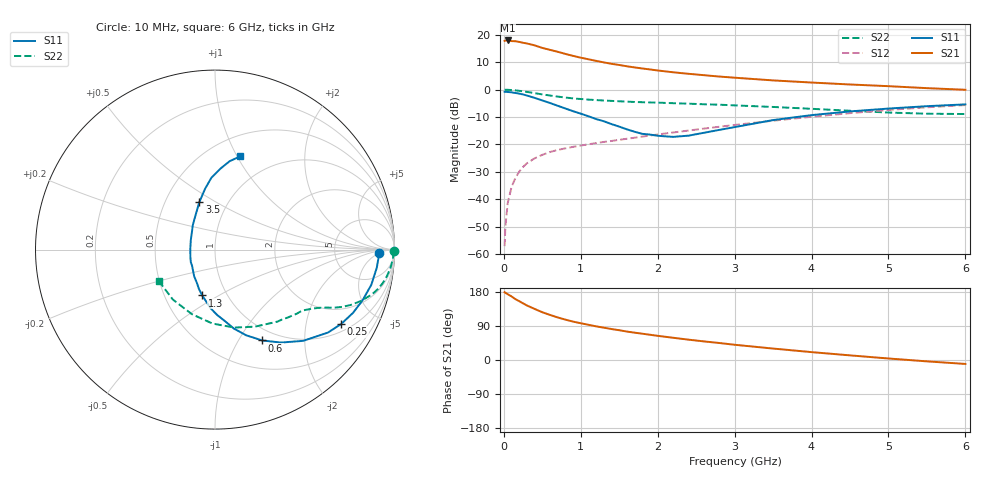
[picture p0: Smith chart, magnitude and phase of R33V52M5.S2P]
! SIEMENS Small Signal Semiconductors
! BFR181
! Si NPN RF Bipolar Junction Transistor in SOT23
! VCE = 3.5 V  IC = 2.5 mA
! Common Emitter S-Parameters:  May  1996
# GHz  S  MA  R  50
!  f  S11  S21  S12  S22
! GHz  MAG  ANG  MAG  ANG  MAG  ANG  MAG  ANG
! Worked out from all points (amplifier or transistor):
!   36 points, 10 MHz to 6 GHz, reference 50 ohm
!   highest |S21| = 17.9 dB at 50 MHz (marker M1)
!   |S21| within 3 dB of that: start of sweep to 539.6 MHz
!   unconditionally stable (mu >= 1): 1.481 GHz to 3.267 GHz
!   at 250 MHz: K = 0.27, MSG = 22.6 dB, |S12| = -28.2 dB
!   at 1.4 GHz: K = 0.98, MSG = 14.1 dB, |S12| = -18.7 dB
!   at 6 GHz: K = 0.86, MSG = 2.8 dB, |S12| = -5.6 dB
!   S11 on the Smith chart (normalised r, x): 10 MHz: 20, -5; 250 MHz: 1.29, -3.19; 600 MHz: 0.84, -1.26; 1.3 GHz: 0.77, -0.42; 3.5 GHz: 0.74, +0.42; 6 GHz: 0.70, +1.03
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0.01  0.9119 -1.3  7.759 178.8  0.0014 87.9  0.9964 -0.6
0.02  0.9127 -2.6  7.836 177.3  0.0032 86.0  0.9944 -1.3
0.05  0.907 -6.4  7.879 173.7  0.0085 87.3  0.9925 -3.0
0.1  0.8926 -12.7  7.675 167.8  0.0168 83.1  0.9829 -5.9
0.15  0.8693 -19.0  7.636 160.6  0.0244 79.0  0.9695 -8.8
0.25  0.8162 -30.5  7.149 149.5  0.0389 72.0  0.9327 -13.7
0.3  0.7808 -36.3  6.94 143.9  0.0455 70.3  0.91 -15.9
0.4  0.7069 -46.0  6.409 134.8  0.0559 65.5  0.8619 -19.4
0.5  0.6347 -54.7  5.761 126.0  0.0647 62.2  0.8183 -22.1
0.6  0.57 -62.6  5.31 119.0  0.0729 59.8  0.7805 -24.1
0.7  0.508 -70.0  4.897 112.3  0.0795 58.2  0.7468 -25.6
0.8  0.453 -76.5  4.475 106.5  0.085 57.0  0.7174 -26.8
0.9  0.4044 -81.8  4.124 101.3  0.0905 56.1  0.6929 -27.8
1.1  0.3272 -94.4  3.574 92.9  0.1007 56.1  0.658 -29.6
1.3  0.265 -105.7  3.136 85.3  0.1114 56.0  0.6337 -31.3
1.7  0.1707 -135.6  2.541 72.1  0.1328 57.4  0.5955 -34.7
2.2  0.1377 177.3  2.072 58.7  0.1654 58.0  0.5661 -40.4
2.8  0.1843 132.1  1.732 44.9  0.2104 57.0  0.5314 -49.0
3.5  0.2785 108.3  1.473 30.2  0.2714 53.5  0.4832 -62.7
4.5  0.4007 92.9  1.241 12.2  0.3723 44.8  0.4121 -92.0
5.5  0.4993 80.6  1.064 -3.6  0.4764 32.3  0.3641 -130.0
6  0.5387 74.8  0.994 -10.4  0.5234 25.1  0.3591 -150.9
